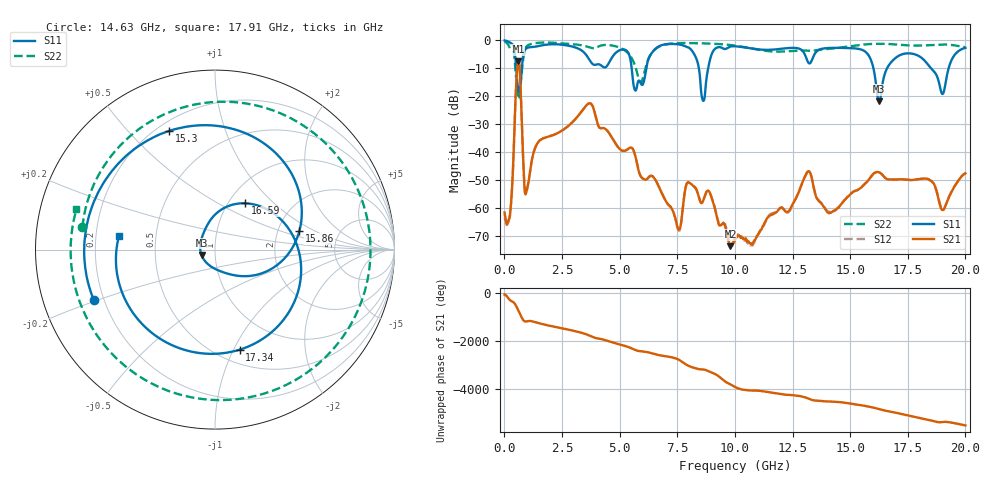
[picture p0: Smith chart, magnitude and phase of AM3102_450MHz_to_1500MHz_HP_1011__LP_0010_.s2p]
!Agilent Technologies,E8364B,MY43040894,A.07.50.67
!Agilent E8364B: A.07.50.67
!Date: Thursday, January 11, 2018 06:23:26
!Correction: S11(Full 2 Port(1,2))
!S21(Full 2 Port(1,2))
!S12(Full 2 Port(1,2))
!S22(Full 2 Port(1,2))
!S2P File: Measurements: S11, S21, S12, S22:
# Hz S  dB  R 50
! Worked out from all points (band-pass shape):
!   1601 points, 10 MHz to 20 GHz, reference 50 ohm
!   highest |S21| = -7.54 dB at 609.7 MHz (marker M1); lowest = -73.7 dB at 9.805 GHz (marker M2)
!   |S21| within 3 dB of the highest: 553.5 MHz to 666.6 MHz (113.1 MHz wide, 18.5 % of centre)
!   lowest |S11| = -21.8 dB at 16.25 GHz (marker M3), VSWR 1.18, Z = 42.9 - j2.59 ohm
!   |S11| at or under -10 dB: 5.521 GHz to 6.157 GHz (635.3 MHz wide, 10.9 % of centre); 16.01 GHz to 16.6 GHz (592.6 MHz wide, 3.63 % of centre); 18.51 GHz to 19.27 GHz (766.7 MHz wide, 4.06 % of centre)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
!   |S22| runs from -21.0 to -0.4 dB; largest |S21 - S12| = 0.0011
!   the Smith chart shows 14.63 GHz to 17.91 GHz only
!   S11 on the Smith chart (normalised r, x): 14.63 GHz: 0.16, -0.19; 15.3 GHz: 0.25, +0.66; 15.86 GHz: 2.63, +0.72; 16.59 GHz: 1.19, +0.68; 17.34 GHz: 0.64, -1.06; 17.91 GHz: 0.30, +0.06
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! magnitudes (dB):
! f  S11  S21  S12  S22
! 10 MHz  -0.1  -61.7  -63.5  -0.4
! 259.9 MHz  -0.9  -61.2  -61.6  -3.2
! 609.7 MHz  -17.8  -7.5  -7.5  -20.8
! 959.5 MHz  -2.9  -54.1  -54.2  -2.2
! 3.346 GHz  -3.6  -25.5  -25.5  -1.8
! 5.695 GHz  -18.0  -41.9  -41.9  -9.8
! 6.682 GHz  -2.2  -52.1  -52.0  -2.4
! 7.556 GHz  -1.4  -67.8  -68.0  -1.0
! 8.618 GHz  -21.6  -57.6  -57.4  -1.1
! 9.805 GHz  -2.2  -73.7  -73.2  -1.7
! 10.01 GHz  -2.1  -71.7  -70.3  -1.9
! 13.34 GHz  -7.1  -49.5  -49.5  -3.8
! 14.63 GHz  -2.7  -58.6  -58.4  -2.5
! 15.3 GHz  -3.0  -53.7  -53.7  -1.8
! 15.86 GHz  -6.3  -49.3  -49.4  -1.3
! 16.25 GHz  -21.8  -47.3  -47.3  -1.2
! 16.59 GHz  -10.2  -49.7  -49.7  -1.3
! 16.68 GHz  -9.0  -49.8  -49.9  -1.3
! 17.34 GHz  -4.8  -49.8  -49.8  -1.7
! 17.91 GHz  -5.4  -49.8  -49.8  -1.9
! 19.01 GHz  -19.2  -60.8  -60.8  -1.5
! 20 GHz  -2.7  -47.6  -47.7  -2.4
